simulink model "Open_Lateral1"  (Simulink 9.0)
settings: Solver=ode45  StartTime=0.0  StopTime=100  RelTol=1e-3  EnableMultiTasking=on
InitFcn:
  | init_lat;
undefined symbols (not defined in the file or in its folder): Al, Bl, Cl, Dl, Kpr

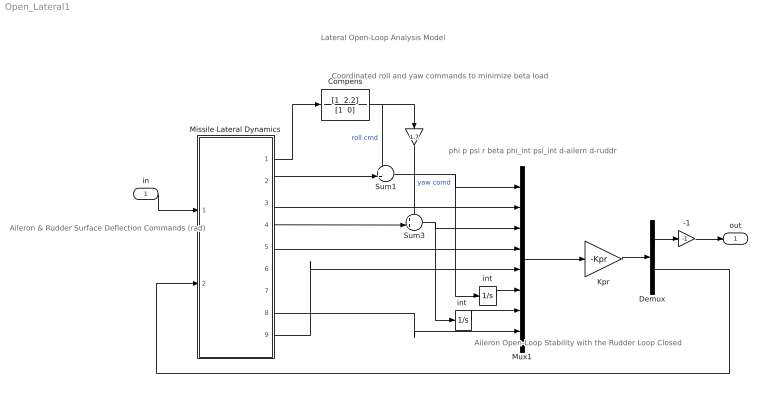
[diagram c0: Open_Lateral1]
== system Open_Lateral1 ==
  note: phi p psi r beta phi_int psi_int d-ailern d-ruddr
  note: Aileron & Rudder Surface Deflection Commands (rad)
  note: Coordinated roll and yaw commands to minimize beta load
  note: Lateral Open-Loop Analysis Model
  note: Aileron Open-Loop Stability with the Rudder Loop Closed
  in : Inport
  " " : Gain  Gain=1.7
  -1 : Gain  Gain=-1
  Compens : TransferFcn  Numerator="[1  2.2]"  Denominator="[1  0]"
  Demux : Demux  Outputs=2
  Kpr : Gain  Gain=-Kpr  Multiplication=Matrix(K*u)
  Missile Lateral Dynamics : Subsystem
  Mux1 : Mux  Inputs=[1, 1, 1, 1, 1, 1, 1, 2]
  Sum1 : Sum  Inputs=++|
  Sum3 : Sum  Inputs=++|
  int : Integrator
  "int " : Integrator
  out : Outport
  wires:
  Missile Lateral Dynamics/3(p) -> Mux1/2
  Missile Lateral Dynamics/5(r) -> Mux1/4
  Sum1/1 -> Mux1/1, int/1
  Missile Lateral Dynamics/2(phi) -> Sum1/2
  Missile Lateral Dynamics/1(" Head") -> Compens/1
  int/1 -> Mux1/6
  Compens/1 -> " "/1, Sum1/1  "roll cmd"
  Missile Lateral Dynamics/4(psi) -> Sum3/2
  Sum3/1 -> Mux1/3, "int "/1
  "int "/1 -> Mux1/7
  " "/1 -> Sum3/1  "yaw comd"
  Mux1/1 -> Kpr/1
  Kpr/1 -> Demux/1
  -1/1 -> out/1
  Missile Lateral Dynamics/8(aeros) -> Mux1/8
  Missile Lateral Dynamics/9(beta-meas) -> Mux1/5
  Demux/1 -> -1/1
  in/1 -> Missile Lateral Dynamics/1(ailer)
  Demux/2 -> Missile Lateral Dynamics/2(ruddr)

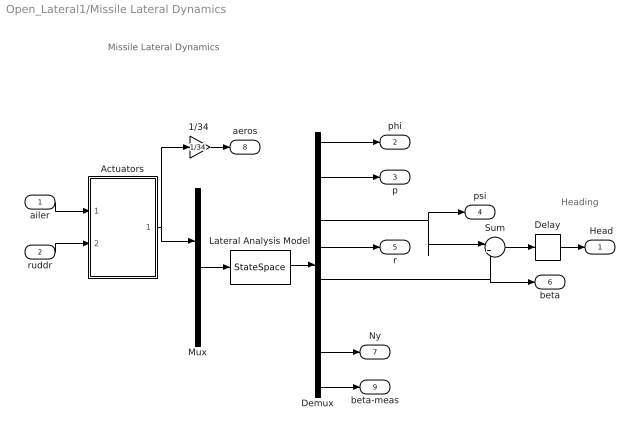
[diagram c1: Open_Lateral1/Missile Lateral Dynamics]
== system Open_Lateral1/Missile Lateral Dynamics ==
  note: Heading
  note: Missile Lateral Dynamics
  ailer : Inport
  ruddr : Inport  Port=2
  "1/34 " : Gain  Gain=1/34
  Actuators : Subsystem
  Delay : TransportDelay  DelayTime=0.5  PadeOrder=2
  Demux : Demux  Outputs=8
  Lateral Analysis Model : StateSpace  A=Al  B=Bl  C=Cl  D=Dl  InitialCondition=0
  Mux : Mux  Inputs=[2, 1]
  Sum : Sum  Inputs=|++
  " Head" : Outport
  phi : Outport  Port=2
  p : Outport  Port=3
  psi : Outport  Port=4
  r : Outport  Port=5
  beta : Outport  Port=6
  Ny : Outport  Port=7
  aeros : Outport  Port=8
  beta-meas : Outport  Port=9
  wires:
  Mux/1 -> Lateral Analysis Model/1
  Demux/1 -> phi/1
  Demux/2 -> p/1
  Demux/4 -> r/1
  Demux/3 -> psi/1, Sum/1
  Demux/5 -> beta/1, Sum/2
  Actuators/1("delo ") -> "1/34 "/1, Mux/1
  Sum/1 -> Delay/1
  ailer/1 -> Actuators/1(dailer)
  ruddr/1 -> Actuators/2(drudr)
  Demux/7 -> Ny/1
  Demux/8 -> beta-meas/1
  Lateral Analysis Model/1 -> Demux/1
  Delay/1 -> " Head"/1
  "1/34 "/1 -> aeros/1

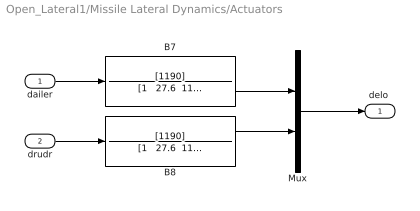
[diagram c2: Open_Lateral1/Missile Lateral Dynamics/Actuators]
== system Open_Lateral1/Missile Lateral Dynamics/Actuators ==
  dailer : Inport
  drudr : Inport  Port=2
  B7 : TransferFcn  Numerator=[1190]  Denominator="[1   27.6  1190]"
  B8 : TransferFcn  Numerator=[1190]  Denominator="[1   27.6  1190]"
  Mux : Mux  Inputs=2
  "delo " : Outport
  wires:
  Mux/1 -> "delo "/1
  B7/1 -> Mux/1
  B8/1 -> Mux/2
  drudr/1 -> B8/1
  dailer/1 -> B7/1
